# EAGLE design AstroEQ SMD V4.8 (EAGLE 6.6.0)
REVISION: V4.8
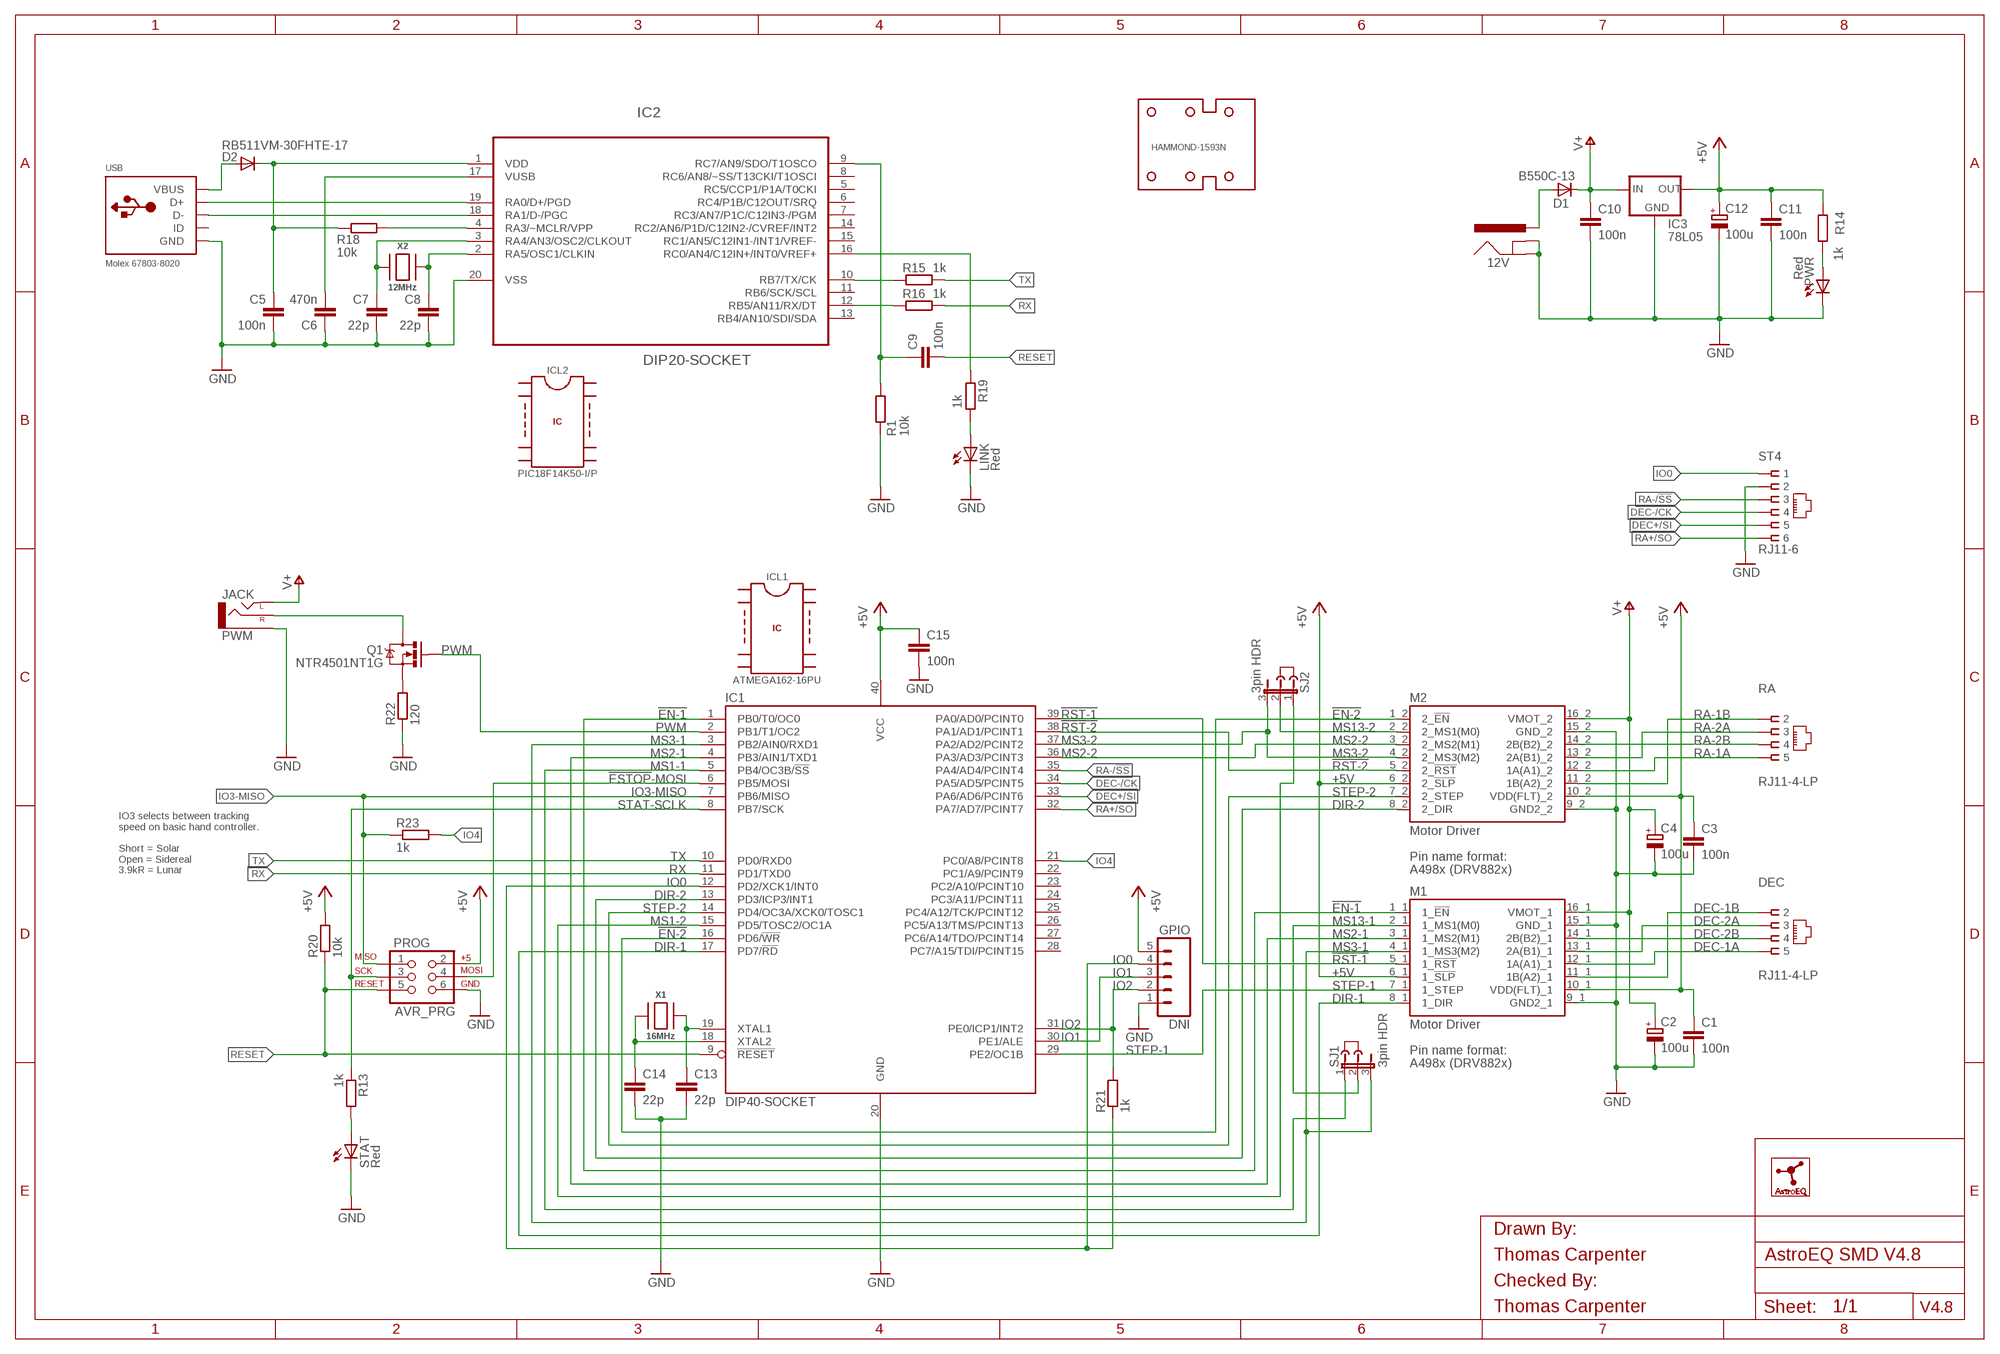
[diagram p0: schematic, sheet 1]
FRAME1 (A3L-LOC): CHECKED_BY: Thomas Carpenter; DRAWN_BY: Thomas Carpenter

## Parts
12V  POWER_JACKPTH  [POWER_JACK_PTH]
C1  100n  C-EUC0603  [C0603]
C2  100u  CPOL-EUD  [PANASONIC_D]
C3  100n  C-EUC0603  [C0603]
C4  100u  CPOL-EUD  [PANASONIC_D]
C5  100n  C-EUC0603  [C0603]
C6  470n  C-EUC0603  [C0603]
C7  22p  C-EUC0603  [C0603]
C8  22p  C-EUC0603  [C0603]
C9  100n  C-EUC0603  [C0603]
C10  100n  C-EUC0603  [C0603]
C11  100n  C-EUC0603  [C0603]
C12  100u  CPOL-EUD  [PANASONIC_D]
C13  22p  C-EUC0603  [C0603]
C14  22p  C-EUC0603  [C0603]
C15  100n  C-EUC0603  [C0603]
D1  B550C-13  DIODE-SMC  [SMC]
D2  RB511VM-30FHTE-17  DIODESOD  [SOD-323]
DEC  RJ11-4-LP  [RJ11-NO_SHIELD-4-LP]
GPIO  DNI  M05PTH  [1X05]
HAMMOND-1593N  HAMMOND-1593N-4HOLE  [HAMMOND-1593N4HOLES]
IC1  DIP40-SOCKET  ATMEGA162-16PU  [DIL40]
IC2  DIP20-SOCKET  PIC18F14K50-I/P-SKT  [DIL20-SKT]
IC3  78L05  V_REG_78XX-SOT89  [SOT89]
ICL1  ATMEGA162-16PU  IC  [IC]
ICL2  PIC18F14K50-I/P  IC  [IC]
J2  DNI  JUMPER  [JUMP]
J3  DNI  JUMPER  [JUMP]
LINK  Red  LED-1206-SIDE  [SML1206-SIDE]
LOGO1  DNI  ASTROEQ5MM  [ASTROEQ-SMALL]
M1  Motor Driver  A4983-DUAL-HV  [CARRIER-HV-DUAL]
M2  Motor Driver  A4983-DUAL-LV  [CARRIER-LV-DUAL]
PROG  AVR_PRG  AVR_SPI_PRG_6PTH  [2X3]
PWM  JACK  AUDIO-JACKPTH  [AUDIO-JACK]
PWR  Red  LED-1206-SIDE  [SML1206-SIDE]
Q1  NTR4501NT1G  MOSFET-NCHANNELSMD  [SOT23-3]
R1  10k  R-EU_R0603  [R0603]
R13  1k  R-EU_R0603  [R0603]
R14  1k  R-EU_R0603  [R0603]
R15  1k  R-EU_R0603  [R0603]
R16  1k  R-EU_R0603  [R0603]
R18  10k  R-EU_R0603  [R0603]
R19  1k  R-EU_R0603  [R0603]
R20  10k  R-EU_R0603  [R0603]
R21  1k  R-EU_R0603  [R0603]
R22  120  R-EU_R0805  [R0805]
R23  1k  R-EU_R0603  [R0603]
RA  RJ11-4-LP  [RJ11-NO_SHIELD-4-LP]
SJ1  3pin HDR  JP2E  [JP2]
SJ2  3pin HDR  JP2E  [JP2]
ST4  RJ11-6  RJ11-LP  [RJ11-NO_SHIELD-LP]
STAT  Red  LED-1206-SIDE  [SML1206-SIDE]
USB  Molex 67803-8020  USBMINIAB  [USB-MINIAB]
X1  16MHz  XTALNX5032  [NX5032]
X2  12MHz  XTALNX5032  [NX5032]

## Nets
!EN-1: IC1.1(PB0/T0/OC0) M2.1_1(1_!EN)
!EN-2: IC1.16(PD6/!WR) M2.1_2(2_!EN)
!ESTOP!-MOSI: IC1.6(PB5/MOSI) PROG.4
!RST-1: IC1.39(PA0/AD0/PCINT0) M2.5_1(1_!RST)
!RST-2: IC1.38(PA1/AD1/PCINT1) M2.5_2(2_!RST)
+5V: C1.1 C3.1 C11.1 C12.+ C15.1 GPIO.5 IC1.40(VCC) IC3.1(OUT) M1.10_1(VDD(FLT)_1) M1.10_2(VDD(FLT)_2) M2.6_1(1_!SLP) M2.6_2(2_!SLP) PROG.2 R14.1 R20.2
AVROSC1: C13.1 IC1.19(XTAL1) X1.P$2
AVROSC2: C14.1 IC1.18(XTAL2) X1.P$1
D_N [usbdat]: IC2.18(RA1/D-/PGC) USB.D-
D_P [usbdat]: IC2.19(RA0/D+/PGD) USB.D+
DEC+/SI: IC1.33(PA6/AD6/PCINT6) ST4.5
DEC-1A: DEC.5 M1.12_1(1A(A1)_1)
DEC-1B: DEC.2 M1.11_1(1B(A2)_1)
DEC-2A: DEC.3 M1.13_1(2A(B1)_1)
DEC-2B: DEC.4 M1.14_1(2B(B2)_1)
DEC-/CK: IC1.34(PA5/AD5/PCINT5) ST4.4
DIR-1: IC1.17(PD7/!RD) M2.8_1(1_DIR)
DIR-2: IC1.13(PD3/ICP3/INT1) M2.8_2(2_DIR)
DTR: C9.1 IC2.9(RC7/AN9/SDO/T1OSCO) R1.1
GND: 12V.GND 12V.GNDBREAK C1.2 C2.- C3.2 C4.- C5.2 C6.1 C7.2 C8.2 C10.2 C11.2 C12.- C13.2 C14.2 C15.2 GPIO.1 IC1.20(GND) IC2.20(VSS) IC3.2(GND) IC3.4(GND) LINK.C LINK.E(C) M1.9_1(GND2_1) M1.9_2(GND2_2) M1.15_1(GND_1) M1.15_2(GND_2) PROG.6 PWM.SLEEVE PWR.C PWR.E(C) R1.2 R22.1 ST4.2 STAT.C STAT.E(C) USB.GND USB.GND1(GND) USB.GND2(GND) USB.GND3(GND) USB.GND4(GND)
IO0: GPIO.4 IC1.12(PD2/XCK1/INT0) R21.1 ST4.1
IO1: GPIO.3 IC1.30(PE1/ALE)
IO2: GPIO.2 IC1.31(PE0/ICP1/INT2) R21.2
IO3-MISO: IC1.7(PB6/MISO) PROG.1 R23.1
IO4: IC1.21(PC0/A8/PCINT8) R23.2
MCLR: IC2.4(RA3/~MCLR/VPP) R18.1
MS1-1: IC1.5(PB4/OC3B/!SS) SJ1.1
MS1-2: IC1.15(PD5/TOSC2/OC1A) SJ2.1
MS2-1: IC1.4(PB3/AIN1/TXD1) M2.3_1(1_MS2(M1))
MS2-2: IC1.36(PA3/AD3/PCINT3) M2.3_2(2_MS2(M1))
MS3-1: IC1.3(PB2/AIN0/RXD1) M2.4_1(1_MS3(M2)) SJ1.3
MS3-2: IC1.37(PA2/AD2/PCINT2) M2.4_2(2_MS3(M2)) SJ2.3
MS13-1: M2.2_1(1_MS1(M0)) SJ1.2
MS13-2: M2.2_2(2_MS1(M0)) SJ2.2
PWM: IC1.2(PB1/T1/OC2) Q1.1(G)
PWM-ILIM: Q1.2(S) R22.2
PWM-OD: PWM.RING(RIGHT) Q1.3(D)
PWRLED: PWR.A R14.2
RA+/SO: IC1.32(PA7/AD7/PCINT7) ST4.6
RA-1A: M1.12_2(1A(A1)_2) RA.5
RA-1B: M1.11_2(1B(A2)_2) RA.2
RA-2A: M1.13_2(2A(B1)_2) RA.3
RA-2B: M1.14_2(2B(B2)_2) RA.4
RA-/!SS: IC1.35(PA4/AD4/PCINT4) ST4.3
RESET: C9.2 IC1.9(!RESET) PROG.5 R20.1
RX: IC1.11(PD1/TXD0) R16.1
RX(USB): IC2.12(RB5/AN11/RX/DT) R16.2
STAT-SCLK: IC1.8(PB7/SCK) PROG.3 R13.1
STATLED: R13.2 STAT.A
STEP-1: IC1.29(PE2/OC1B) M2.7_1(1_STEP)
STEP-2: IC1.14(PD4/OC3A/XCK0/TOSC1) M2.7_2(2_STEP)
TX: IC1.10(PD0/RXD0) R15.1
TX(USB): IC2.10(RB7/TX/CK) R15.2
USBLED: LINK.A R19.1
USBOSC1: C8.1 IC2.2(RA5/OSC1/CLKIN) X2.P$2
USBOSC2: C7.1 IC2.3(RA4/AN3/OSC2/CLKOUT) X2.P$1
USBSTAT: IC2.16(RC0/AN4/C12IN+/INT0/VREF+) R19.2
V+: C2.+ C4.+ C10.1 D1.C IC3.3(IN) M1.16_1(VMOT_1) M1.16_2(VMOT_2) PWM.TIP(LEFT)
VBUS: D2.2(A) USB.VBUS
VIN: 12V.PWR D1.A
VPIC: C5.1 D2.1(C) IC2.1(VDD) R18.2
VUSB: C6.2 IC2.17(VUSB)
Unconnected: IC1.22(PC1/A9/PCINT9) IC1.23(PC2/A10/PCINT10) IC1.24(PC3/A11/PCINT11) IC1.25(PC4/A12/TCK/PCINT12) IC1.26(PC5/A13/TMS/PCINT13) IC1.27(PC6/A14/TDO/PCINT14) IC1.28(PC7/A15/TDI/PCINT15) IC2.5(RC5/CCP1/P1A/T0CKI) IC2.6(RC4/P1B/C12OUT/SRQ) IC2.7(RC3/AN7/P1C/C12IN3-/PGM) IC2.8(RC6/AN8/~SS/T13CKI/T1OSCI) IC2.11(RB6/SCK/SCL) IC2.13(RB4/AN10/SDI/SDA) IC2.14(RC2/AN6/P1D/C12IN2-/CVREF/INT2) IC2.15(RC1/AN5/C12IN1-/INT1/VREF-) USB.ID

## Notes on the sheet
- IO3 selects between tracking
  speed on basic hand controller.
  
  Short = Solar
  Open = Sidereal
  3.9kR = Lunar

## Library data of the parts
12V = SparkFun:POWER_JACK: Power Jack This is the standard 5.5mm barrel jack for power. The PTH is the most common, proven, reliable, footprint. All others are experimental. The Slot footprint only works if the mill layer is transmitted to the PCB fab house so be warned. Spark Fun Electronics SKU : PRT-00119. Mating wall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; MF: MULTICOMP; MPN: MJ-179PH; OC_FARNELL: 1737246
C1 C3 C5 C9-C11 C15 = rcl:C-EU: CAPACITOR, European symbol; MF: MULTICOMP; MPN: MC0603F104Z250CT; OC_FARNELL: 1759038
C2 C4 C12 = rcl:CPOL-EU: POLARIZED CAPACITOR, European symbol; MF: WURTH ELEKTRONIK; MPN: 865080545012; OC_FARNELL: 2466321
C6 = rcl:C-EU: CAPACITOR, European symbol; MF: MULTICOMP; MPN: MC0603F474Z160CT; OC_FARNELL: 1759021
C7 C8 C13 C14 = rcl:C-EU: CAPACITOR, European symbol; MF: MULTICOMP; MPN: MC0603N220J500CT; OC_FARNELL: 1759057
D1 = diode:DIODE-: DIODE; MF: DIODES INC.; MPN: B550C-13-F; OC_FARNELL: 1858608
D2 = SparkFun:DIODE: Diode; MF: ROHM; MPN: RB511VM-30FHTE-17; OC_FARNELL: 2581544
DEC RA = con-tycoelectronics:RJ11-4; MF: MOLEX; MPN: 95501-2641; OC_FARNELL: 1560166
GPIO = SparkFun:M05: Header 5 Standard 5-pin 0.1" header. Use with straight break away headers (SKU : PRT-00116), right angle break away headers (PRT-00553), swiss pins (PRT-00743), machine pins (PRT-00117), and female headers (PRT-00115). Molex polarized connector foot print use with SKU : PRT-08230 with associated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; OC_FARNELL: unknown
HAMMOND-1593N = holes:HAMMOND-1593N; MF: HAMMOND; MPN: 1593NBK; OC_FARNELL: 9287566
IC1 = atmel:ATMEGA162: 8-bit RISC MICROCONTROLLER 16K Bytes internal flash program memory 1K Bytes internal SRAM Upto 64K Bytes optional external memory space 512 Bytes EEPROM Two 8-bit timers Two 16-bit timers Dual programmable serial USARTs Master/Slave serial SPI interface Source: ATMEGA162_DIP40.lbr; MF: MULTICOMP; MPN: 2227MC-40-06-05-F1; OC_FARNELL: 1103855
IC2 = microchip:PIC18F14K50: USB Flash Microcontrollers; MF: MULTICOMP
IC3 = SparkFun:V_REG_78XX: Voltage Regulator Standard 7805 5V regulator. IGO (Input Ground Output). Spark Fun Electronics SKU : COM-00107; MF: STMICROELECTRONICS; MPN: L78L05ACUTR; OC_FARNELL: 1366573
ICL1 = ic-package:IC; MF: ATMEL; MPN: ATMEGA162-16PU; OC_FARNELL: 9171169
ICL2 = ic-package:IC; MF: MICROCHIP; MPN: PIC18F14K50-I/P; OC_FARNELL: 1648501
J2 J3 = jumper:JUMPER: JUMPER header; MF: 3M; MPN: 969102-0000-DA; OC_FARNELL: 2579814
LINK PWR STAT = led:LED: LED; MF: WURTH ELEKTRONIK; MPN: 155124RS73200; OC_FARNELL: 2322101
LOGO1 = CompanyLogos:ASTROEQ; OC_FARNELL: unknown
M1 = A4983Carrier:A4983-DUAL-HV; MF: SAMTEC; MPN: CES-116-01-T-S; OC_FARNELL: 1667522
M2 = A4983Carrier:A4983-DUAL-LV; MF: SAMTEC; MPN: CES-116-01-T-S; OC_FARNELL: 1667522
PROG = SparkFun:AVR_SPI_PRG_6: AVR ISP 6 Pin This is the reduced ISP connector for AVR programming. Common on Arduino. This footprint will take up less PCB space and can be used with a 10-pin to 6-pin adapter such as SKU: BOB-08508; MF: HARWIN; MPN: M20-9980346; OC_FARNELL: 1022231
PWM = SparkFun:AUDIO-JACK: 3.5mm Audio Jack Simple 3.5mm common PCB mount audio jack. SKU: PRT-08032; MF: CLIFF ELECTRONIC COMPONENTS; MPN: FC68131; OC_FARNELL: 2518188
Q1 = SparkFun:MOSFET-NCHANNEL; MF: ON SEMICONDUCTOR; MPN: NTR4501NT1G; OC_FARNELL: 1431305
R1 R18 R20 = rcl:R-EU_: RESISTOR, European symbol; MF: MULTICOMP; MPN: MCWR06X1002FTL; OC_FARNELL: 2447230
R13-R16 R19 R21 R23 = rcl:R-EU_: RESISTOR, European symbol; MF: MULTICOMP; MPN: MCWR06X1001FTL; OC_FARNELL: 2447272
R22 = rcl:R-EU_: RESISTOR, European symbol; MF: MULTICOMP; MPN: MCWR08X1200FTL; OC_FARNELL: 2447561
SJ1 SJ2 = jumper:JP2E: JUMPER; MF: HARWIN; MPN: M20-9990345.; OC_FARNELL: 1022248
ST4 = con-tycoelectronics:RJ11: CORCOM Modular RJ Jacks No Shield Source: www.tycoelectronics.com .. ENG_DS_1654001_1099_RJ_L_0507.pdf; MF: MOLEX; MPN: 95501-2661; OC_FARNELL: 1536490
USB = adafruit:USB: USB Connectors USBMINIB - Surface Mount Female Mini-B USB Connector 4UConnector: 06564 By microbuilder.eu Thru-hole RA Female Mini-B USB Connector 4UConnector: 18732 By ladyada.net; MF: MOLEX; MPN: 67803-8020; OC_FARNELL: 1355761
X1 = adafruit:XTAL: Low cost SMT crystals, no capacitors included; MF: TXC; MPN: 7A-16.000MAAJ-T; OC_FARNELL: 1841946
X2 = adafruit:XTAL: Low cost SMT crystals, no capacitors included; MF: TXC; MPN: 7A-12.000MAAJ-T; OC_FARNELL: 1841940

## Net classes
1 power: width 0.61 mm, drill 0.711 mm, clearance 0.203 mm
2 gnd: width 0.305 mm, drill 0.711 mm, clearance 0.203 mm
3 usbvcc: width 0.508 mm, drill 0.711 mm, clearance 0.203 mm
4 usbdat: width 0.406 mm, clearance 0.152 mm

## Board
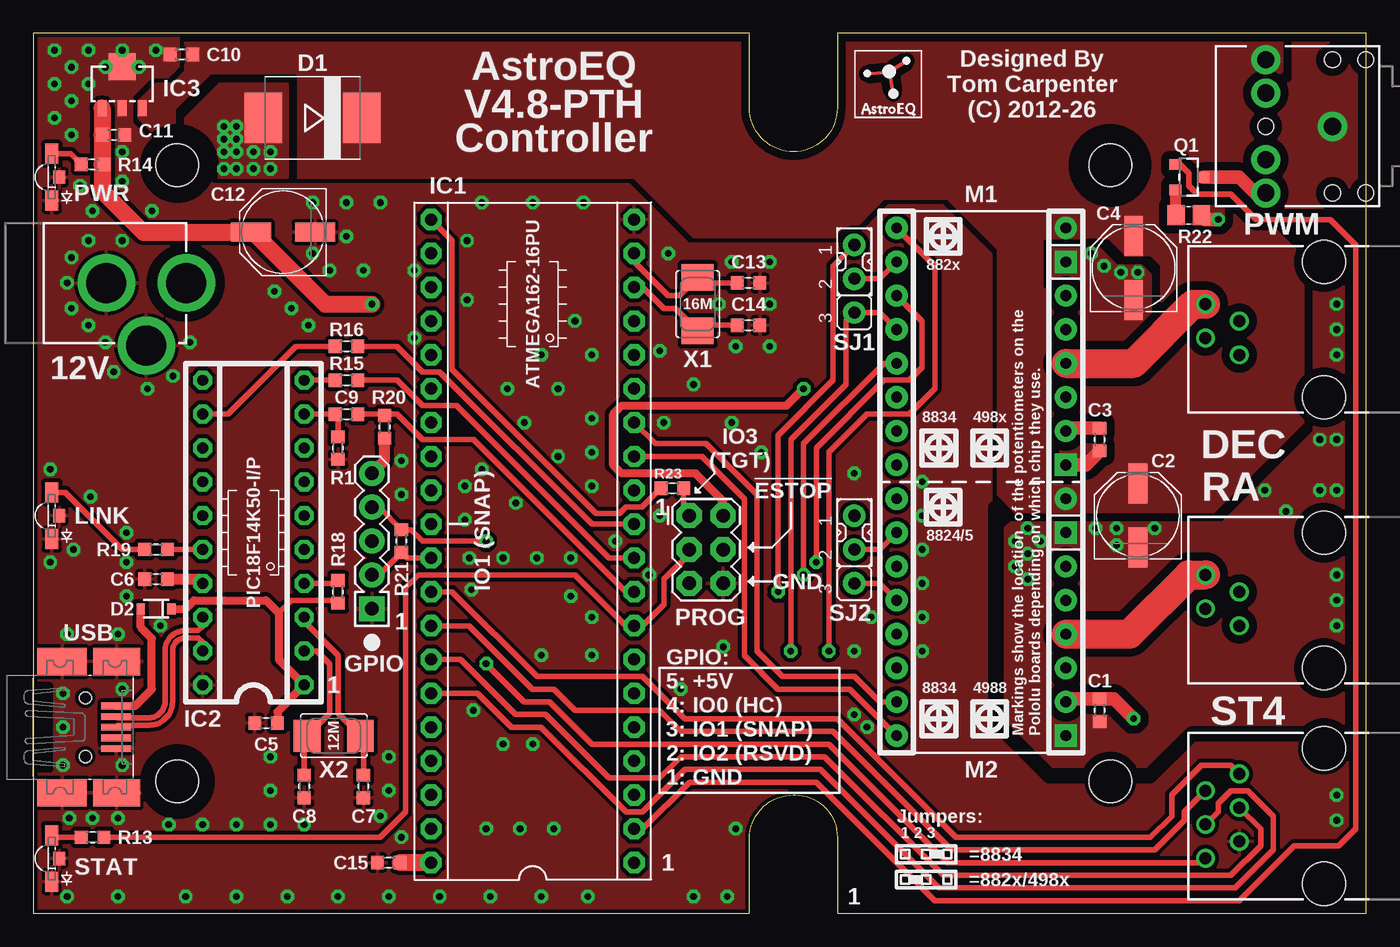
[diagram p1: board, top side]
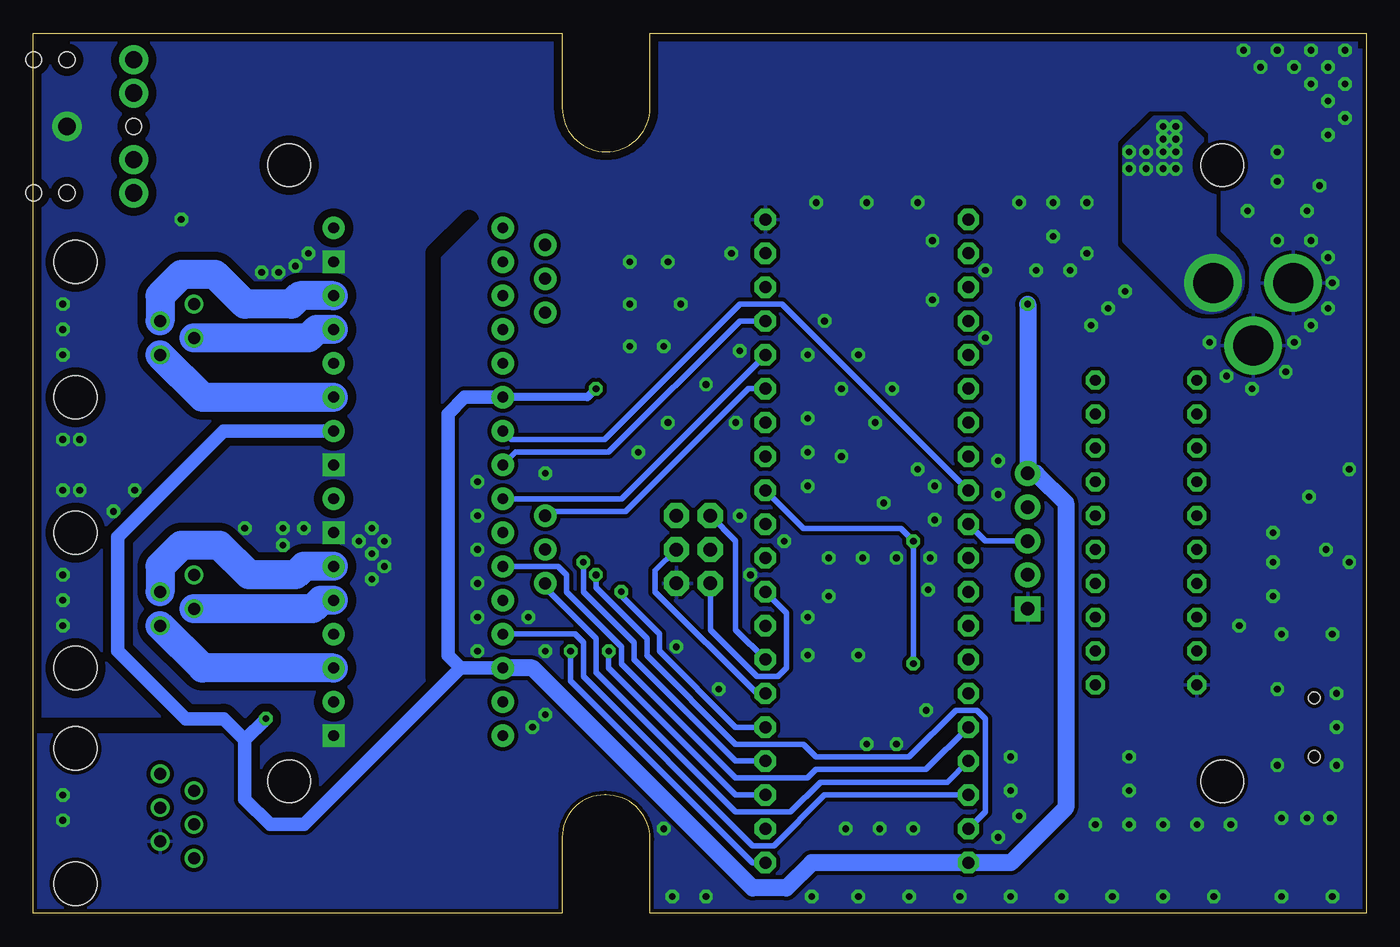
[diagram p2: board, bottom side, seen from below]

Size 100 x 66.04 mm. Coordinates in mm from the lower left corner, seen from the top.
Outline: 57.02,8.89 57.15,8.89
Copper layers (1*16): Top 0.035mm / dielectric 1.5mm / Bottom 0.035mm
Design rules "pcbtrain *": minimum track width 0.2mm, minimum drill 0.4mm, track to track 6mil, track to pad 6mil, pad to pad 6mil, via to via 6mil, smd to smd 0mil, copper to edge 10mil, drill to drill 0.2mm, minimum pad ring 10mil, minimum via ring 10mil, stop-mask expansion 0.125mm, vias tented up to drill 0.75mm, thermal gap 10mil
tKeepout: area 78.3,7.4 to 83.3,12.4; area 78.3,53.6 to 83.3,58.6; area 8.3,7.4 to 13.3,12.4; area 8.3,53.6 to 13.3,58.6
bKeepout: area 78.3,7.4 to 83.3,12.4; area 78.3,53.6 to 83.3,58.6; area 8.3,7.4 to 13.3,12.4; area 8.3,53.6 to 13.3,58.6
tRestrict: area 78.3,53.6 to 83.3,58.6; area 8.3,7.4 to 13.3,12.4; area 8.3,53.6 to 13.3,58.6; area 9,44.8 to 13.9,49.8; 7 lines
bRestrict: 3 lines

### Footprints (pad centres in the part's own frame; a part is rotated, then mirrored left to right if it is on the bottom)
POWER_JACK_PTH = drill 2.997 pad 4.318: GND 0,7.7; GNDBREAK 4.7,10.7; PWR 0,13.7
C0603 = smd 0.95 x 1: 1 -0.85,0; 2 0.85,0
PANASONIC_D = smd 3 x 1.4: + 2.4,0; - -2.4,0
SMC = smd 2.8 x 3.8: A 3.7,0; C -3.7,0
SOD-323 = smd 0.63 x 0.83: 1 -1.15,0; 2 1.15,0
RJ11-NO_SHIELD-4-LP = drill 0.9 pad 1.4: 2 -1.905,6.35; 3 -0.635,8.89; 4 0.635,6.35; 5 1.905,8.89 | hole 3.251: -5.08,0; 5.08,0
1X05 = drill 1.016 pad 1.88 square: 1 -5.08,0 | drill 1.016 pad 1.88: 2 -2.54,0; 3 0,0; 4 2.54,0; 5 5.08,0
HAMMOND-1593N4HOLES = hole 3.2: 10.795,9.906; 10.795,56.134; 80.797,9.906; 80.797,56.134
DIL40 = drill 0.9 pad 1.6 octagon: 1 -24.13,-7.62; 2 -21.59,-7.62; 3 -19.05,-7.62; 4 -16.51,-7.62; 5 -13.97,-7.62; 6 -11.43,-7.62; 7 -8.89,-7.62; 8 -6.35,-7.62; 9 -3.81,-7.62; 10 -1.27,-7.62; 11 1.27,-7.62; 12 3.81,-7.62; 13 6.35,-7.62; 14 8.89,-7.62; 15 11.43,-7.62; 16 13.97,-7.62; 17 16.51,-7.62; 18 19.05,-7.62; 19 21.59,-7.62; 20 24.13,-7.62; 21 24.13,7.62; 22 21.59,7.62; 23 19.05,7.62; 24 16.51,7.62; 25 13.97,7.62; 26 11.43,7.62; 27 8.89,7.62; 28 6.35,7.62; 29 3.81,7.62; 30 1.27,7.62; 31 -1.27,7.62; 32 -3.81,7.62; 33 -6.35,7.62; 34 -8.89,7.62; 35 -11.43,7.62; 36 -13.97,7.62; 37 -16.51,7.62; 38 -19.05,7.62; 39 -21.59,7.62; 40 -24.13,7.62
DIL20-SKT = drill 0.813 pad 1.422 octagon: 1 -3.81,11.43; 2 -3.81,8.89; 3 -3.81,6.35; 4 -3.81,3.81; 5 -3.81,1.27; 6 -3.81,-1.27; 7 -3.81,-3.81; 8 -3.81,-6.35; 9 -3.81,-8.89; 10 -3.81,-11.43; 11 3.81,-11.43; 12 3.81,-8.89; 13 3.81,-6.35; 14 3.81,-3.81; 15 3.81,-1.27; 16 3.81,1.27; 17 3.81,3.81; 18 3.81,6.35; 19 3.81,8.89; 20 3.81,11.43
SOT89 = smd 0.65 x 1.2: 1 -1.5,-1.8; 2 0,-1.8; 3 1.5,-1.8 | smd 2 x 2: 4 0,1.3
SML1206-SIDE = smd 1.5 x 1: A 1.75,0; C -1.75,0 | smd 1 x 0.9: E 0,-0.55
CARRIER-HV-DUAL = drill 0.813 pad 1.676 square: 9_1 -1.27,0; 9_2 19.05,0; 15_1 -16.51,0; 15_2 3.81,0 | drill 0.813 pad 1.676: 10_1 -3.81,0; 10_2 16.51,0; 11_1 -6.35,0; 11_2 13.97,0; 12_1 -8.89,0; 12_2 11.43,0; 13_1 -11.43,0; 13_2 8.89,0; 14_1 -13.97,0; 14_2 6.35,0; 16_1 -19.05,0; 16_2 1.27,0
CARRIER-LV-DUAL = drill 0.813 pad 1.676: 1_1 -19.05,0; 1_2 1.27,0; 2_1 -16.51,0; 2_2 3.81,0; 3_1 -13.97,0; 3_2 6.35,0; 4_1 -11.43,0; 4_2 8.89,0; 5_1 -8.89,0; 5_2 11.43,0; 6_1 -6.35,0; 6_2 13.97,0; 7_1 -3.81,0; 7_2 16.51,0; 8_1 -1.27,0; 8_2 19.05,0
2X3 = drill 1.016 pad 1.88 octagon: 1 -2.54,-1.27; 2 -2.54,1.27; 3 0,-1.27; 4 0,1.27; 5 2.54,-1.27; 6 2.54,1.27
AUDIO-JACK = drill 1.3 pad 2.184: RING 5,5; RSH 5,2.5; SLEEVE 0,0; TIP 5,-5; TSH 5,-2.5 | hole 1.2: 0,5; -2.5,5; -2.5,-5; 0,-5; 5,0
SOT23-3 = smd 0.8 x 0.9: 1 -0.95,-1; 2 0.95,-1; 3 0,1.1
R0603 = smd 0.95 x 1: 1 -0.85,0; 2 0.85,0
R0805 = smd 1.3 x 1.5: 1 -0.95,0; 2 0.95,0
JP2 = drill 0.914 pad 1.676: 1 -2.54,0; 2 0,0; 3 2.54,0
RJ11-NO_SHIELD-LP = drill 0.9 pad 1.4: 1 -3.175,8.89; 2 -1.905,6.35; 3 -0.635,8.89; 4 0.635,6.35; 5 1.905,8.89; 6 3.175,6.35 | hole 3.251: -5.08,0; 5.08,0
USB-MINIAB = smd 0.5 x 2.25: D+ 0,2.225; D- -0.8,2.225; GND 1.6,2.225; ID 0.8,2.225; VBUS -1.6,2.225 | smd 2.05 x 3.7: GND1 -4.925,-1.85; GND4 4.925,-1.85 | smd 2.05 x 3.5: GND2 -4.925,2.25; GND3 4.925,2.25 | hole 0.9: -2.2,-0.1; 2.2,-0.1
NX5032 = smd 2 x 2.4: P$1 2,0; P$2 -2,0

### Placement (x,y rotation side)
12V  -2.22,47.31 270 top
C1  80.01,15.24 270 top
C2  82.87,29.84 90 top
C3  80.01,35.56 270 top
C4  82.55,48.42 90 top
C5  17.46,14.29 180 top
C6  9.21,25.08 0 top
C7  24.77,9.53 270 top
C8  20.32,9.53 270 top
C9  23.5,37.47 0 top
C10  11.11,64.45 180 top
C11  6.03,58.42 0 top
C12  18.73,51.12 180 top
C13  53.66,47.31 0 top
C14  53.66,44.13 0 top
C15  26.67,3.81 180 top
D1  20.95,59.69 180 top
D2  9.21,22.86 180 top
DEC  96.84,43.81 90 top
GPIO  25.4,27.94 90 top
HAMMOND-1593N  0,0 0 top
IC1  37.47,27.94 90 top
IC2  16.51,28.57 180 top
IC3  6.67,62.23 0 top
ICL1  37.47,45.72 180 top
ICL2  16.51,28.57 180 top
J2  61.59,28.57 0 top
J3  61.59,48.9 0 top
LINK  1.38,29.84 90 top
LOGO1  61.59,59.69 0 top
M1  77.47,32.38 270 top
M2  64.77,32.38 270 top
PROG  50.48,27.3 270 top
PWM  97.47,59.05 180 top
PWR  1.38,55.24 90 top
Q1  86.68,55.24 270 top
R1  22.86,34.92 270 top
R13  4.45,5.71 180 top
R14  4.45,56.2 180 top
R15  23.5,40.01 180 top
R16  23.5,42.55 180 top
R18  22.86,24.13 270 top
R19  9.21,27.3 0 top
R20  26.35,36.51 270 top
R21  27.62,27.94 270 top
R22  86.68,52.39 180 top
R23  47.94,31.91 180 top
RA  96.84,23.5 90 top
SJ1  61.59,47.62 270 top
SJ2  61.59,27.3 270 top
ST4  96.84,7.3 90 top
STAT  1.38,4.13 90 top
USB  4,13.97 270 top
X1  49.85,45.72 270 top
X2  22.54,13.34 0 top

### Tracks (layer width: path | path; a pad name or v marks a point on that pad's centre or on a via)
!EN-1  (via drill 0.5)
  Top 0.406: M2.1_1 67.63,48.58 67.63,39.37 65.72,37.47 62.55,37.47 59.69,34.61 v59.69,19.68
  Bottom 0.406: IC1.1 46.04,3.81 59.69,17.46 v59.69,19.68
!EN-2
  Bottom 0.406: M2.1_2 55.88,31.11 IC1.16
!ESTOP!-MOSI
  Bottom 0.406: IC1.6 45.72,16.51 53.34,24.13 53.34,25.72 PROG.4
!RST-1  (via drill 0.5)
  Top 0.406: M2.5_1 63.82,41.27 57.78,35.24 v57.78,25.4
  Bottom 0.406: IC1.39 28.57,7.62 28.57,14.61 29.21,15.24 30.8,15.24 34.29,11.75 41.27,11.75 42.23,12.7 47.31,12.7 53.98,19.37 53.98,20.64 57.78,24.45 v57.78,25.4
!RST-2
  Bottom 0.406: IC1.38 40.64,8.89 44.45,5.08 46.04,5.08 58.74,17.78 58.74,20.32 59.37,20.95 M2.5_2
+5V  (via drill 0.5, 0.5 pad 0.25)
  Top 0.406: R14.1 5.17,56.2 | C11.1 5.17,58.42
  Top 0.6: PROG.2 51.75,30.96
  Top 0.61: 51.75,30.96 49.69,33.02 44.13,33.02 43.5,33.66 43.5,37.47 44.13,38.1 56.52,38.1 v57.78,39.37
  Top 0.813: GPIO.5 26.35,33.97 R20.2
  Top 1.016: M1.10_1 77.69,36.41 C3.1 | M1.10_2 77.69,16.09 C1.1 81.06,16.09 v82.55,14.61
  Top 1.27: IC3.1 5.17,58.42 5.17,56.2 5.17,54.2 8.26,51.12 C12.+ 16.51,51.12 21.91,45.72 v25.4,45.72 | IC1.40 C15.1
  Bottom 0.61: v57.78,39.37 58.42,38.73 M2.6_1
  Bottom 1.016: M1.10_1 85.72,36.2 93.66,28.26 93.66,19.68 88.58,14.61 85.72,14.61 84.14,13.02 | v82.55,14.61 84.14,13.02 | 84.14,13.02 84.14,8.57 82.23,6.67 79.69,6.67 67.94,18.41 | 67.94,18.41 M2.6_2 | 67.94,18.41 68.9,19.37 68.9,37.47 67.63,38.73 M2.6_1
  Bottom 1.27: v25.4,45.72 GPIO.5 24.77,33.02 22.54,30.8 22.54,7.94 26.67,3.81 IC1.40 41.59,3.81 43.5,1.91 46.04,1.91 62.55,18.41 M2.6_2
AVROSC1
  Top 0.406: IC1.19 45.09,48.9 47.62,46.35 48.48,46.35 X1.P$2 50.26,47.31 C13.1
AVROSC2
  Top 0.406: IC1.18 45.72,46.99 47.31,45.4 48.16,45.4 X1.P$1 50.26,44.13 C14.1
D_N
  Top 0.406: IC2.18 12.7,21.55 12.38,21.23 11.43,21.23 arc90 9.88,19.68 9.88,15.88 arc-90 8.69,14.68 6.32,14.68 USB.D-
D_P
  Top 0.406: IC2.19 12.7,20.36 12.38,20.68 11.43,20.68 arc90 10.44,19.68 10.44,15.88 arc-90 8.69,14.12 6.38,14.12 USB.D+
DEC+/SI
  Top 0.406: IC1.33 32.7,21.59 37.47,16.83 39.05,16.83 40.64,15.24 46.99,15.24 48.58,13.65 60.01,13.65 68.9,4.76 84.14,4.76 86.36,6.99 86.36,7.62 ST4.5
DEC-1A
  Top 2.184: M1.12_1 82.55,41.27 87,45.72 DEC.5
DEC-1B
  Bottom 2.184: DEC.2 87.31,38.73 M1.11_1
DEC-2A
  Bottom 2.184: M1.13_1 78.74,43.81 79.38,43.18 DEC.3
DEC-2B
  Bottom 2.184: M1.14_1 80.01,46.35 80.64,45.72 84.14,45.72 86.36,47.94 88.9,47.94 90.49,46.35 DEC.4
DEC-/CK
  Top 0.406: IC1.34 32.07,19.05 36.2,14.92 38.42,14.92 43.18,10.16 46.99,10.16 48.58,11.75 59.37,11.75 68.26,2.86 89.85,2.86 92.08,5.08 92.08,6.35 ST4.4
DIR-1
  Bottom 0.406: IC1.17 46.99,44.45 56.83,34.61 63.82,34.61 M2.8_1
DIR-2
  Top 0.406: M2.8_2 61.28,16.83 55.88,16.83 53.34,19.37 53.34,31.11 50.16,34.29 IC1.13
DTR
  Top 0.406: IC2.9 C9.1 22.86,37.25 R1.1
GND  (via drill 0.5)
  Top 1.016: C3.2 78.95,33.66 M1.9_1 | v88.9,52.07 87.94,52.07 R22.1
  other vias: 6.67,57.15 6.67,54.93 8.89,52.7 1.59,64.77 6.67,64.77 4.13,64.77 1.59,62.23 4.13,62.23 1.59,59.69 2.86,60.96 2.86,63.5 5.4,63.5 4.45,52.7 6.67,50.48 3.49,54.61 7.94,63.5 9.21,64.77 2.86,58.42 79.38,49.53 82.87,48.1 81.6,48.1 80.33,48.58 79.69,28.89 81.28,28.89 84.14,28.89 81.28,27.62 96.52,35.56 97.79,35.56 96.52,31.75 97.79,31.75 97.79,45.72 97.79,41.91 97.79,43.81 97.79,23.5 97.79,21.59 97.79,25.4 97.79,8.89 97.79,6.99 74.61,28.89 74.61,26.99 74.61,25.08 73.66,27.94 73.66,26.04 75.56,27.94 92.39,31.75 93.98,30.16 2.22,16.51 2.22,11.11 2.22,13.97 6.67,16.83 6.67,11.11 2.7,7.14 6.35,7.14 6.35,20.95 2.54,20.95 9.53,21.59 6.99,26.35 6.99,23.81 4.29,31.27 6.99,28.57 1.27,33.34 1.27,26.35 3.02,27.3 2.54,1.27 6.35,1.27 11.43,1.27 15.24,1.27 19.05,1.27 22.86,1.27 26.67,1.27 30.48,1.27 34.29,1.27 38.1,1.27 41.59,1.27 49.53,1.27 52.07,1.27 4.13,50.48 2.86,49.21 2.86,45.4 4.13,44.13 5.4,42.86 11.75,42.86 10.48,40.32 8.57,39.37 6.03,40.64 2.54,47.31 20.64,44.13 19.37,45.4 18.1,46.67 20.95,49.53 22.23,48.26 24.77,48.26 20.95,53.34 23.5,53.34 23.5,50.8 26.04,53.34 33.66,53.34 37.47,53.34 41.27,53.34 47.62,49.53 51.44,45.72 55.24,45.72 55.24,48.9 55.24,42.55 52.7,42.55 52.39,48.9 20.32,6.67 17.78,9.21 17.78,11.75 26.67,11.75 26.67,9.21 27.62,5.71 4.45,7.14 17.78,6.67 15.24,6.67 12.7,6.67 10.16,6.67 26.04,7.3 36.83,36.83 39.37,39.37 35.56,39.37 38.1,41.91 40.64,44.45 41.91,41.91 33.02,15.24 35.24,12.7 37.47,12.7 61.59,14.92 61.59,19.68 62.55,13.97 66.67,19.68 66.67,22.23 66.67,24.77 66.67,27.3 66.67,29.84 66.67,32.38 62.87,22.23 33.97,6.35 36.51,6.35 39.05,6.35 54.61,34.61 52.39,36.83 49.53,39.69 46.99,42.23 61.59,33.02 48.58,16.83 51.75,20 41.91,32.07 41.91,34.61 41.91,37.15 47.31,36.83 32.86,24.29 40.32,23.81 38.1,19.37 41.91,19.37 41.91,22.23 27.62,33.97 27.62,31.43 35.24,26.67 40.32,26.67 32.38,29.53 32.38,32.07 33.66,33.34 36.2,30.8 39.37,34.29 37.78,26.67 32.7,26.67 46.2,25.4 52.7,6.35 28.57,43.18 32.54,46.04 28.57,48.26 32.54,50.48 46.99,29.84 43.66,27.94
  pour Top (isolate 0.305, rank 3): -1.27,66.99 72.07,66.99 72.07,14.29 76.2,10.16 82.55,10.16 87.63,15.24 102.3,15.24 102.3,-0.95 -1.27,-0.95
  pour Bottom (isolate 0.305, rank 3): -1.27,64.77 35.56,64.77 46.99,53.34 65.15,53.34 69.91,48.58 69.85,16.51 80.01,6.35 81.92,6.35 84.14,8.57 84.14,13.02 85.09,13.97 101.66,14.29 101.66,-0.95 -1.27,-0.95
  pour Top (isolate 0.305, rank 3, no thermals): -1.27,67.31 -1.27,57.47 11.43,57.47 11.43,67.31
  pour Top (isolate 0.61, rank 3, no thermals): 71.12,67.31 71.12,9.21 101.6,9.21 101.6,67.31
  pour Top (isolate 0.61, no thermals): 76.52,49.85 80.01,49.85 81.28,48.58 83.19,48.58 83.82,47.94 83.82,41.91 76.52,41.91
  pour Bottom (isolate 0.61, rank 3): -2.54,68.58 -2.54,-2.54 102.87,-2.54 102.87,68.58
  pour Bottom (isolate 0.61, rank 3, no thermals): 71.12,66.04 71.12,7.94 101.6,7.94 101.6,66.04
IO0  (via drill 0.5)
  Top 0.406: GPIO.4 25.93,30.48 R21.1 28.36,28.79 29.21,27.94 v33.97,27.94 | ST4.1 87.63,3.81 68.58,3.81 59.69,12.7 41.91,12.7 38.73,15.88 36.83,15.88 v33.97,18.73
  Bottom 0.406: v33.97,18.73 v33.97,27.94 34.92,28.89 42.23,28.89 IC1.12
IO1
  Bottom 0.406: IC1.30 28.57,27.94 GPIO.3
IO2
  Top 0.406: IC1.31 28.04,26.67 R21.2 25.93,25.4 GPIO.2
IO3-MISO
  Top 0.406: PROG.1 48.79,30.27 R23.1
  Bottom 0.406: IC1.7 47.31,21.27 47.31,27.94 PROG.1
IO4
  Top 0.406: R23.2 45.66,30.48 44.45,30.48 43.97,30 42.23,30 31.43,40.8 31.43,50.48 IC1.21
MCLR
  Top 0.406: IC2.4 22.64,24.77 R18.1
MS1-1  (via drill 0.5)
  Top 0.406: v55.88,24.13 55.88,35.88 60.01,40.01 60.01,48.58 SJ1.1
  Bottom 0.406: IC1.5 47.31,13.97 53.02,19.68 53.02,20.95 55.88,23.81 v55.88,24.13
MS1-2
  Bottom 0.406: SJ2.1 61.28,30.16 55.56,30.16 46.35,39.37 IC1.15
MS2-1  (via drill 0.5)
  Top 0.406: v58.74,26.35 58.74,34.92 63.82,40.01 65.72,40.01 66.67,40.96 66.67,44.45 M2.3_1
  Bottom 0.406: IC1.4 47.31,11.43 54.93,19.05 54.93,20.32 58.74,24.13 v58.74,26.35
MS2-2
  Bottom 0.406: M2.3_2 60.64,26.04 60.01,25.4 60.01,24.13 55.88,20 55.88,18.73 47.31,10.16 41.91,10.16 41.27,10.79 33.02,10.79 IC1.36
MS3-1  (via drill 0.5)
  Top 0.406: M2.4_1 63.5,45.09 SJ1.3 60.96,44.45 60.96,39.69 56.83,35.56 v56.83,19.68
  Bottom 0.406: IC1.3 47.31,8.89 56.83,18.41 v56.83,19.68
MS3-2
  Top 0.406: M2.4_2 63.5,24.77 SJ2.3
  Bottom 0.406: IC1.37 31.43,9.84 40.96,9.84 43.18,7.62 47.31,7.62 57.78,18.1 57.78,20.64 61.59,24.45 SJ2.3
MS13-1
  Top 0.406: M2.2_1 63.5,47.62 SJ1.2
MS13-2
  Top 0.406: M2.2_2 63.5,27.3 SJ2.2
PWM
  Top 0.406: Q1.1 86.05,56.2 86.68,55.56 86.68,54.61 87.31,53.98 89.85,53.98 91.76,52.07 97.31,52.07 99.22,50.16 99.22,6.35 97.95,5.08 94.61,5.08 90.49,0.95 67.63,0.95 58.74,9.84 49.21,9.84 45.72,6.35 IC1.2
PWM-ILIM
  Top 0.406: 85.68,52.44 R22.2
  Top 0.813: Q1.2 85.68,52.44
PWM-OD
  Top 1.016: PWM.RING 91.68,54.05 90.49,55.24 Q1.3
PWRLED
  Top 0.406: PWR.A 2.8,56.99 R14.2
RA+/SO
  Top 0.406: IC1.32 31.43,24.13 37.78,17.78 45.72,17.78 48.9,14.61 60.33,14.61 69.22,5.71 83.82,5.71 85.41,7.3 85.41,8.89 87.63,11.11 89.85,11.11 ST4.6
RA-1A
  Top 2.184: M1.12_2 82.23,20.95 86.68,25.4 RA.5
RA-1B
  Bottom 2.184: M1.11_2 87.31,18.41 RA.2
RA-2A
  Bottom 2.184: M1.13_2 78.42,23.5 79.06,22.86 RA.3
RA-2B
  Bottom 2.184: M1.14_2 79.69,26.04 80.33,25.4 83.82,25.4 86.04,27.62 88.9,27.62 90.49,26.04 RA.4
RA-/!SS
  Top 0.406: IC1.35 33.34,16.51 35.88,13.97 38.1,13.97 44.45,7.62 45.72,7.62 48.9,10.79 59.05,10.79 67.94,1.91 90.17,1.91 93.03,4.76 93.03,7.3 91.12,9.21 89.85,9.21 88.9,8.26 88.9,7.62 ST4.3
RESET
  Top 0.406: C9.2 26.35,37.47 | 26.35,37.47 27.3,37.47 29.21,35.56 33.02,35.56 44.45,24.13 IC1.9 | R20.1 26.35,37.47
  Bottom 0.406: IC1.9 43.5,22.54 43.5,18.41 44.13,17.78 45.72,17.78 49.21,21.27 PROG.5
RX
  Top 0.406: R16.1 27.3,42.55 29.21,40.64 30.48,40.64 41.91,29.21 IC1.11
RX(USB)
  Top 0.406: IC2.12 14.61,37.47 19.68,42.55 R16.2
STAT-SCLK
  Top 0.406: R13.1 26.04,5.71 27.94,7.62 27.94,24.45 28.89,25.4 40.64,25.4 44.45,21.59 IC1.8 45.72,21.59 47.31,23.18 47.31,25.08 49.21,26.99 PROG.3
STATLED
  Top 0.406: STAT.A 1.58,5.88 1.75,5.71 R13.2
STEP-1
  Bottom 0.406: IC1.29 43.81,45.72 46.99,45.72 57.15,35.56 64.14,35.56 M2.7_1
STEP-2
  Top 0.406: IC1.14 46.67,35.24 50.48,35.24 54.29,31.43 54.29,19.68 56.2,17.78 61.59,17.78 63.5,15.88 M2.7_2
TX
  Top 0.406: R15.1 27.3,40.01 29.21,38.1 31.75,38.1 43.18,26.67 IC1.10
TX(USB)
  Top 0.406: IC2.10 R15.2
USBLED
  Top 0.406: LINK.A 2.38,31.59 6.67,27.3 R19.1
USBOSC1
  Top 0.406: IC2.2 21.27,19.68 22.23,18.73 22.23,15.02 X2.P$2 20.32,13.11 C8.1
USBOSC2
  Top 0.406: IC2.3 20.32,21.91 22.86,19.37 22.86,15.02 X2.P$1 24.77,13.11 C7.1
USBSTAT
  Top 0.406: R19.2 IC2.16
V+
  pour Top (isolate 0.61, rank 2, no thermals): 93.66,67.31 11.43,67.31 11.43,63.18 10.48,62.23 9.21,62.23 7.94,60.96 7.94,59.69 12.38,55.24 45.09,55.24 49.53,50.8 60.96,50.8 63.82,53.66 68.58,53.66 72.39,49.85 72.39,31.43 73.66,30.16 88.58,30.16 95.25,36.83 95.25,49.21 91.44,53.02 91.44,60.96 93.66,63.18
VBUS
  Top 0.61: USB.VBUS 7.63,15.57 8.89,16.83 8.89,20.64 8.06,21.47 D2.2
VIN  (via drill 0.5)
  other vias: 15.24,55.88 17.78,55.88 14.29,57.15 15.24,57.15 16.51,55.88 17.78,57.15 15.24,59.05 14.29,58.1 16.51,57.15 15.24,58.1 14.29,55.88 14.29,59.05
  pour Top (isolate 0.61, no thermals): 13.97,62.23 19.05,62.23 19.05,55.24 11.43,55.24 11.43,59.69
  pour Bottom (isolate 0.61, no thermals): 11.43,57.15 13.97,59.69 15.88,59.69 18.1,57.47 18.1,50.48 13.34,45.72 arc-180 10.16,49.53 11.43,50.8
VPIC
  Top 0.406: R18.2 22.64,23.5 19.37,23.5 18.41,22.54
  Top 0.61: D2.1 11.43,22.86 12.06,23.5 17.46,23.5 18.41,22.54 18.41,19.05 IC2.1 18.31,15.14 C5.1
VUSB
  Top 0.813: C6.2 12.38,25.08 IC2.17

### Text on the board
tPlace: 1 | 1 | 1 | Markings show the location of the potentiometers on the | Pololu boards depending on which chip they use. | Jumpers: | 1 2 3 | 1 | =8834 | =882x/498x | 1
tNames: Designed By | AstroEQ | Tom Carpenter | V4.8-PTH | (C) 2012-26 | Controller | 16M | IO3 / (TGT) | !ESTOP! | IO1 (SNAP) | GND | GPIO: / 5: +5V / 4: IO0 (HC) / 3: IO1 (SNAP) / 2: IO2 (RSVD) / 1: GND | 12M
Reference: This board design is for purchased AstroEQ controllers. | Due to the large number of surface mount components, this board / is not designed to be DIY-ed. | For DIY, use "AstroEQ PTH V4.8"

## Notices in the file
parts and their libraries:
SparkFun: Licensing: CC v3.0 Share-Alike You are welcome to use this library for commercial purposes.
